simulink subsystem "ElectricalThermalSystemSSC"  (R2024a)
settings: Solver=VariableStepAuto  StartTime=0.0  StopTime=10.0  RelTol=1e-3
undefined symbols (not defined in the file): coolant_pipe_D, coolant_valve_D_ratio_max, coolant_valve_D_ratio_min, coolant_valve_displacement, EnvAirTemp, EnvGrvty, PlantThrEstCmpPwr, PlntThrChArea, PlntThrFanMaxSpd, PlntThrFanMechEff, PlntThrFanVolEff, PlntThrHeaterMaxPwr, PlntThrPipeArea, PlntThrPipeDia, PlntThrPmpMaxSpd, PlntThrRadRamEff, PlntThrRefrigAinit, PlntThrTankArea, PlntThrTankVol, PlntThrValDisp, PlntThrValDratioMax, PlntThrValDratioMin, PlntThrValSplMax, ThrmEM1, ThrmEM2, ThrmEM3, ThrmEM4
libraries: fl_lib x148, nesl_utility x61, SimscapeFluids_lib x25, autolibutils x12
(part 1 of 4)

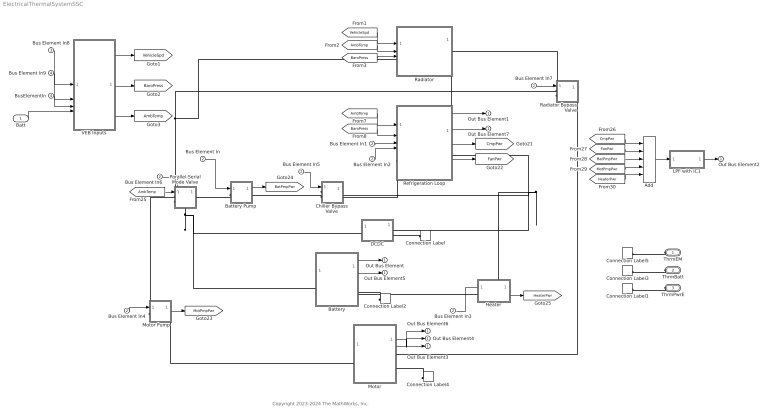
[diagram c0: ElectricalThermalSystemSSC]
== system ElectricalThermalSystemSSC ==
  note: Copyright 2023-2024 The MathWorks, Inc.
  Batt : Inport
  Bus Element In{,1..7} (8 alike) : Inport  Port=2
  Bus Element In8 : Inport  Port=3
  Bus Element In9 : Inport  Port=4
  BusElementIn : Inport  Port=4
  Add : Sum  Inputs=+++++
  Battery : Subsystem  Tag=PublishSubsystem
  Battery Pump : Subsystem  Tag=PublishSubsystem
  Chiller Bypass Valve : Subsystem  Tag=PublishSubsystem
  Connection Label : ConnectionLabel  Label=ThrmPwrE
  Connection Label1 : ConnectionLabel  Label=ThrmPwrE
  Connection Label2 : ConnectionLabel  Label=ThrmBatt
  Connection Label3 : ConnectionLabel  Label=ThrmBatt
  Connection Label4 : ConnectionLabel  Label=ThrmEM
  Connection Label5 : ConnectionLabel  Label=ThrmEM
  DCDC : Subsystem  Tag=PublishSubsystem
  Heater : Subsystem  Tag=PublishSubsystem
  LPF with IC1 : Subsystem  mask{wc=10, InitCond=0, dataType=off}
      mask prompts: wc "Cutoff frequency, wc [rad/s]"; InitCond "Initial condition, InitCond [same as u]"; dataType "Enforce same input data type"
  Motor : Subsystem  Tag=PublishSubsystem
  Motor Pump : Subsystem  Tag=PublishSubsystem
  Parallel-Serial Mode Valve : Subsystem  Tag=PublishSubsystem
  Radiator : Subsystem  Tag=PublishSubsystem
  Radiator Bypass Valve : Subsystem  Tag=PublishSubsystem
  Refrigeration Loop : Subsystem  Tag=detailed cycle  Variant=on  VariantControlMode=label  VariantControl=Choice  LabelModeActiveChoice=System Level
  VEB Inputs : Subsystem
  ThrmEM : PMIOPort  Side=Left
  ThrmBatt : PMIOPort  Port=2  Side=Left
  ThrmPwrE : PMIOPort  Port=3  Side=Left
  Out Bus Element{,1..7} (8 alike) : Outport
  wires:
  Add/1 -> LPF with IC1/1(u)
  Battery/1(01) -> Out Bus Element/1
  [VehicleSpd] -> Radiator/1(1)
  [AmbTemp] -> Radiator/2(2)
  [BaroPress] -> Radiator/3(3)
  [AmbTemp] -> Refrigeration Loop/1(AmbTemp)
  [BaroPress] -> Refrigeration Loop/2(BaroPress)
  Refrigeration Loop/1(CondPress) -> Out Bus Element1/1
  Bus Element In1/1 -> Refrigeration Loop/3(CmpCmd)
  Refrigeration Loop/2(ChlrPress) -> Out Bus Element7/1
  Motor/1(01) -> Out Bus Element4/1, Out Bus Element6/1
  Battery/2(02) -> Out Bus Element5/1
  Bus Element In2/1 -> Refrigeration Loop/4(FanCmd)
  Bus Element In3/1 -> Heater/1(1)
  Bus Element In4/1 -> Motor Pump/1(1)
  Bus Element In/1 -> Battery Pump/1(1)
  Bus Element In5/1 -> Chiller Bypass Valve/1(1)
  Bus Element In6/1 -> Parallel-Serial Mode Valve/2(2)
  Bus Element In7/1 -> Radiator Bypass Valve/1(1)
  [AmbTemp] -> Parallel-Serial Mode Valve/1(1)
  Batt/1 -> VEB Inputs/4(Batt)
  VEB Inputs/1(VehicleSpd) -> [VehicleSpd]
  VEB Inputs/3(AmbTemp) -> [AmbTemp]
  VEB Inputs/2(BaroPress) -> [BaroPress]
  Refrigeration Loop/3(CmpPwr) -> [CmpPwr]
  Refrigeration Loop/4(FanPwr) -> [FanPwr]
  Motor Pump/1(2) -> [MotPmpPwr]
  Battery Pump/1(2) -> [BatPmpPwr]
  [CmpPwr] -> Add/1
  [FanPwr] -> Add/2
  [BatPmpPwr] -> Add/3
  [MotPmpPwr] -> Add/4
  LPF with IC1/1(y) -> Out Bus Element2/1
  Heater/1(2) -> [HeaterPwr]
  [HeaterPwr] -> Add/5
  Motor/2(02) -> Out Bus Element3/1
  Bus Element In8/1 -> VEB Inputs/1(VehBody)
  Bus Element In9/1 -> VEB Inputs/2(Press)
  BusElementIn/1 -> VEB Inputs/3(Temp)
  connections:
  Chiller Bypass Valve/RConn1 -- Heater/RConn1 -- DCDC/RConn1 -- Refrigeration Loop/RConn1
  Parallel-Serial Mode Valve/RConn2 -- Battery/LConn1 -- DCDC/LConn1
  Parallel-Serial Mode Valve/LConn2 -- Radiator/LConn1 -- Radiator Bypass Valve/LConn1
  Connection Label/LConn1 -- DCDC/RConn2
  ThrmPwrE/RConn1 -- Connection Label1/LConn1
  Connection Label2/LConn1 -- Battery/RConn2
  ThrmBatt/RConn1 -- Connection Label3/LConn1
  Connection Label4/LConn1 -- Motor/RConn2
  ThrmEM/RConn1 -- Connection Label5/LConn1
  Battery/RConn1 -- Heater/LConn1
  Motor Pump/RConn1 -- Motor/LConn1
  Radiator Bypass Valve/RConn1 -- Motor/RConn1
  Radiator Bypass Valve/LConn2 -- Radiator/RConn1
  Chiller Bypass Valve/LConn1 -- Battery Pump/RConn1
  Refrigeration Loop/LConn1 -- Chiller Bypass Valve/LConn2
  Battery Pump/LConn1 -- Parallel-Serial Mode Valve/RConn1
  Radiator/RConn2 -- Refrigeration Loop/LConn2
  Motor Pump/LConn1 -- Parallel-Serial Mode Valve/LConn1

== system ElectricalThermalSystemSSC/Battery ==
  Batt Cool1 : fl_lib/Thermal/Thermal Elements/Thermal Mass  mass_type=foundation.enum.constant_variable.constant  mass=1 kg  sp_heat=PlntBattCp J/(K*kg)  mass_min=1e-6 kg  num_ports=foundation.enum.numPorts2.two  m_specify=off  m_priority=High  m=1 kg  m_nominal_specify=off  m_nominal_value=1  m_nominal_unit=kg  T_specify=on  T_priority=High  T=EnvAirTemp K  T_nominal_specify=off  T_nominal_value=1  T_nominal_unit=K  Q_specify=off  Q_priority=None  Q=0 W  Q_nominal_specify=off  Q_nominal_value=1  Q_nominal_unit=W
  Coolant Jacket 1 : SimscapeFluids_lib/Thermal Liquid/Pipes & Fittings/Pipe (TL)  dynamic_compressibility=simscape.enum.onoff.on  inertia=simscape.enum.onoff.off  num_segments=1  pipe_length=PlntThrBattJacLen m  cross_section_geometry=fluids.thermal_liquid.pipes_fittings.enum.CrossSectionGeometry.Custom  pipe_diameter=0.1 m  pipe_inner_diameter=0.05 m  pipe_outer_diameter=0.1 m  pipe_width=0.1 m  pipe_height=0.1 m  pipe_major_axis=0.1 m  pipe_minor_axis=0.05 m  pipe_side=0.1 m  pipe_angle=30 deg  area=4*PlntThrChArea m^2  Dh=PlntThrChDia m  elevation_spec=foundation.enum.constant_variable.constant  elevation_gain=0 m  gravity_spec=foundation.enum.constant_variable.constant  g=EnvGrvty m/s^2  pressure_loss_spec=fluids.thermal_liquid.pipes_fittings.enum.PressureLossSpec.Haaland  local_pressure_loss_spec=fluids.thermal_liquid.pipes_fittings.enum.LocalLossSpec.AggregateLength  length_add=0 m  loss_coefficient=0.1  roughness_spec=fluids.thermal_liquid.pipes_fittings.enum.RoughnessSpec.Custom  roughness=1.5e-5 m  Re_friction_TLU=[ 400 1000 1.5e+3 3e+3 4e+3 6e+3 1e+4 2e+4 4e+4 6e+4 1e+5 1e+8 ]  friction_factor_TLU=[ 0.264 0.112 0.07099999999999999 0.0417 0.0387 0.0268 0.025 0.0232 0.0226 0.022 0.0214 0.0214 ]  Re_lam=100  Re_tur=500  shape_factor=64  mdot_nominal=[ 0.1 1 ] kg/s  p_diff_nominal=[ 0.001 0.01 ] MPa  mdot_threshold=1e-6 kg/s  wall_spec=fluids.thermal_liquid.pipes_fittings.enum.wall_spec.rigid  vol_expansion_spec=fluids.thermal_liquid.pipes_fittings.enum.VolumeExpansionSpec.Diameter  area_pressure_gain=1e-6 m^2/MPa  static_pressure_TLU=[.1, 1] MPa  area_pressure_gain_TLU=[1e-05, 1.1e-05] m^2  material_behavior_spec=fluids.thermal_liquid.pipes_fittings.enum.PipeMaterialBehavior.Linear  diameter_pressure_gain=1.2e-6 m/MPa  wall_thickness=0.05 m  elastic_modulus=69 GPa  stress_TLU=[276, 310] MPa  strain_TLU=[.004, .02]  stress_assert_action=simscape.enum.assert.action.none  stress_max=400 MPa  poisson_ratio=0.33  wall_time_constant=0.01 s  thermal_expansion=false  alpha_L_wall=24 um/(deltaK*m)  thermal_expansion_Tref=293.15 K  heat_transfer_spec=fluids.thermal_liquid.pipes_fittings.enum.HeatTransferSpec.DittusBoelter  mdot_nominal_heat=[ 0.1 1 ] kg/s  T_in_nominal=[ 293.15 293.15 ] K  T_out_nominal=[ 300 300 ] K  p_in_nominal_heat=[ 0.101325 0.101325 ] MPa  T_wall_nominal=[ 303.15 303.15 ] K  a_coeff=0.3  b_Re_power=0.8  c_Pr_power=0.33  Nu_lam=3.66  Re_Colburn_TLU=[ 100 150 1000 ]  Colburn_factor_TLU=[ 0.019 0.013 0.002 ]  Re_Nu_TLU=[ 100 150 1000 ]  Pr_Nu_TLU=[ 1 10 ]  Nu_TLU=[ 3.72 4.21; 3.75 4.44; 4.21 7.15 ]  p0_vec=EnvAbsPrs Pa  T0_vec=EnvAirTemp K  mdot0=0.1 kg/s
  Flow Resistance (TL) : fl_lib/Thermal Liquid/Elements/Flow Resistance (TL)  delta_p_nominal=200 Pa  mdot_nominal=0.02 kg/s  area=PlntThrPipeArea m^2  laminar_fraction=1e-3
  S1 : Subsystem
  SC1 : Subsystem
  SC2 : Subsystem
  Simscape Bus2 : SimscapeBus  HierarchyStrings=ThrmBatt1
  B : PMIOPort  Side=Left
  A : PMIOPort  Port=2  Side=Right
  T : PMIOPort  Port=3  Side=Right
  01 : Outport
  02 : Outport  Port=2
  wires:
  S1/1(BattTemp) -> 02/1
  SC1/1(BattCoolTemp) -> 01/1
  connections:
  Batt Cool1/LConn1 -- S1/RConn1
  Batt Cool1/RConn1 -- Simscape Bus2/LConn1
  S1/LConn1 -- Coolant Jacket 1/LConn2
  SC1/LConn1 -- Coolant Jacket 1/LConn1
  A/RConn1 -- SC1/RConn1
  SC2/RConn1 -- Coolant Jacket 1/RConn1
  SC2/LConn1 -- Flow Resistance (TL)/LConn1
  Flow Resistance (TL)/RConn1 -- B/RConn1
  T/RConn1 -- Simscape Bus2/RConn1

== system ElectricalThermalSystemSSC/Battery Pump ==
  1 : Inport
  Battery Pump : SimscapeFluids_lib/Thermal Liquid/Pumps & Motors/Fixed-Displacement Pump (TL)  loss_spec=fluids.thermal_liquid.pumps_motors.enum.LossSpec.TabulatedEfficiency  displacement=PlntThrPmpDisp l/rev  omega_nominal=0.5 * PlntThrPmpMaxSpd rpm  p_nominal=0.1 MPa  mu_nominal=0.9 cP  vol_eff_nominal=PlntThrPmpVolEff  mech_eff_nominal=PlntThrPmpMechEff  no_load_torque=0.03 N*m  p_diff_eff_TLU=[.1, 1, 2] MPa  omega_eff_TLU=[25, 50, 100, 200, 300, 400] rad/s  vol_eff_TLU=[.816, .908, .954, .977, .981, .984; .325, .663, .831, .916, .925, .946; .137, .568, .78, .892, .893, .91]  mech_eff_TLU=[.996, .996, .996, .996, .996, .996; .988, .989, .989, .989, .989, .99; .981, .981, .982, .982, .983, .984]  p_diff_loss_TLU=[.1, 1, 2] MPa  omega_loss_TLU=[25, 50, 100, 200, 300, 400] rad/s  vol_loss_TLU=[.023, .023, .023, .023, .0285, .032; .0844, .0842, .0845, .084, .1125, .108; .1079, .108, .11, .108, .1605, .18] * 1e-3 m^3/s  mech_loss_TLU=[.002, .002, .002, .002, .002, .002; .0607, .0556, .0556, .0556, .0556, .0505; .1937, .1937, .1833, .1833, .1729, .1626] N*m  vol_eff_min=1e-3  vol_eff_max=1  mech_eff_min=1e-3  mech_eff_max=1  pressure_threshold=1e-3 MPa  omega_threshold=10 rad/s  area=PlntThrPipeArea m^2  supplied_range_check=0  pump_mode_check=simscape.enum.assert.action.none
  Ideal Angular Velocity Source : fl_lib/Mechanical/Mechanical Sources/Ideal Angular Velocity Source
  Ideal Rotational Motion Sensor : fl_lib/Mechanical/Mechanical Sensors/Ideal Rotational Motion Sensor  reference=foundation.enum.MeasurementReference.difference  acceleration_port=false  velocity_port=true  position_port=true  wrap_angle=false  offset=0 rad
  Ideal Torque Sensor : fl_lib/Mechanical/Mechanical Sensors/Ideal Torque Sensor
  LPF with IC1 : Subsystem  mask{wc=0.2, InitCond=0, dataType=off}
      mask prompts: wc "Cutoff frequency, wc [rad/s]"; InitCond "Initial condition, InitCond [same as u]"; dataType "Enforce same input data type"
  Max Speed [rpm] : Gain  Gain=PlntThrPmpMaxSpd
  Mechanical Rotational Reference : fl_lib/Mechanical/Rotational Elements/Mechanical Rotational Reference
  Mechanical Rotational Reference1 : fl_lib/Mechanical/Rotational Elements/Mechanical Rotational Reference
  PS Product : fl_lib/Physical Signals/Functions/PS Product
  PS-Simulink Converter : nesl_utility/PS-Simulink Converter  PhysicalDomain=network_engine_domain  SubClassName=ps_output  LeftPortType=input  RightPortType=output  PseudoPeriodic=off  Frequencies=[]  VectorFormat=inherit  Unit=W  AffineConversion=off
  Simulink-PS Converter : nesl_utility/Simulink-PS Converter  PhysicalDomain=network_engine_domain  SubClassName=ps_input  LeftPortType=input  RightPortType=output  PseudoPeriodic=off  Frequencies=[]  NoiseDistribution=none  NoiseParameters=[]  Unit=rpm  AffineConversion=off  FilteringAndDerivatives=provide  SimscapeFilterOrder=1  InputFilterTimeConstant=0.001  UdotUserProvided=0
  A : PMIOPort  Side=Left
  B : PMIOPort  Port=2  Side=Right
  2 : Outport
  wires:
  PS-Simulink Converter/1 -> 2/1
  Max Speed [rpm]/1 -> Simulink-PS Converter/1
  1/1 -> LPF with IC1/1(u)
  LPF with IC1/1(y) -> Max Speed [rpm]/1
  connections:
  Ideal Rotational Motion Sensor/LConn1 -- Ideal Angular Velocity Source/LConn1 -- Ideal Torque Sensor/LConn1
  Ideal Torque Sensor/RConn1 -- Battery Pump/RConn1
  PS Product/LConn1 -- Ideal Rotational Motion Sensor/RConn2
  PS-Simulink Converter/LConn1 -- PS Product/RConn1
  PS Product/LConn2 -- Ideal Torque Sensor/RConn2
  Mechanical Rotational Reference1/LConn1 -- Ideal Rotational Motion Sensor/RConn1
  Battery Pump/LConn2 -- B/RConn1
  Battery Pump/LConn1 -- A/RConn1
  Battery Pump/RConn2 -- Mechanical Rotational Reference/LConn1 -- Ideal Angular Velocity Source/RConn2
  Simulink-PS Converter/RConn1 -- Ideal Angular Velocity Source/RConn1

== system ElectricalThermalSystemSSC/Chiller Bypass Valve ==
  1 : Inport
  Bias : Bias  Bias=-1
  Chiller Bypass Valve : SimscapeFluids_lib/Thermal Liquid/Valves & Orifices/Directional Control Valves/3-Way Directional Valve (TL)  open_orifices_pos=fluids.thermal_liquid.valves.directional_control_valves.enum.OpenOrifices3Way.PA  open_orifices_neg=fluids.thermal_liquid.valves.directional_control_valves.enum.OpenOrifices3Way.AT  area_spec=fluids.thermal_liquid.valves.directional_control_valves.enum.area_spec.identical  valve_spec=fluids.thermal_liquid.valves.enum.orifice_spec.linear  del_S_max=PlntThrValDisp m  area_max=pi * (PlntThrValDratioMax*PlntThrPipeDia)^2 / 4 m^2  del_S_TLU=[0 0.002 0.004 0.007 0.017] m  valve_area_TLU=[1e-09, 2.0352e-07, 4.0736e-05, .00011438, .00034356] m^2  del_S_flow_TLU=[0 0.002 0.004 0.007 0.017] m  p_diff_TLU=[-.1, .3, .5, .7] MPa  vol_flow_TLU=1e-3 * [1.7e-05, 2e-05, 2.6e-05; .0035, .0045, .0053; .7, .9, 1.06; 1.96, 2.5, 3; 6, 7.7, 9.13] m^3/s  mdot_TLU=[-1e-05, 1.7e-05, 2e-05, 2.6e-05; -.002, .0035, .0045, .0053; -.4, .7, .9, 1.06; -1.13, 1.96, 2.5, 3; -3.45, 6, 7.7, 9.13] kg/s  T_ref_in=293.15 K  p_ref_in=0.101325 MPa  area_leak=pi * (PlntThrValDratioMin*PlntThrPipeDia)^2 / 4 m^2  Cd=0.7  Re_c=12  smoothing_factor=0.01  pressure_recovery=simscape.enum.onoff.on  area=pi *PlntThrPipeDia^2 / 4 m^2  S_max_PA=PlntThrValSplMax m  del_S_max_PA=coolant_valve_displacement-(coolant_valve_displacement)*(pi * (coolant_valve_D_ratio_min*coolant_pipe_D)^2 / 4)/(pi * (coolant_valve_D_ratio_max*coolant_pipe_D)^2 / 4) m  area_max_PA=pi * (coolant_valve_D_ratio_max*coolant_pipe_D)^2 / 4 m^2  del_S_TLU_PA=[0 0.002 0.004 0.007 0.017] m  valve_area_TLU_PA=[1e-09, 2.0352e-07, 4.0736e-05, .00011438, .00034356] m^2  del_S_flow_TLU_PA=[0 0.002 0.004 0.007 0.017] m  p_diff_TLU_PA=[-.1, .3, .5, .7] MPa  vol_flow_TLU_PA=1e-3 * [1.7e-05, 2e-05, 2.6e-05; .0035, .0045, .0053; .7, .9, 1.06; 1.96, 2.5, 3; 6, 7.7, 9.13] m^3/s  mdot_TLU_PA=[-1e-05, 1.7e-05, 2e-05, 2.6e-05; -.002, .0035, .0045, .0053; -.4, .7, .9, 1.06; -1.13, 1.96, 2.5, 3; -3.45, 6, 7.7, 9.13] kg/s  S_max_AT=-PlntThrValSplMax m  del_S_max_AT=coolant_valve_displacement-(coolant_valve_displacement)*(pi * (coolant_valve_D_ratio_min*coolant_pipe_D)^2 / 4)/(pi * (coolant_valve_D_ratio_max*coolant_pipe_D)^2 / 4) m  area_max_AT=pi * (coolant_valve_D_ratio_max*coolant_pipe_D)^2 / 4 m^2  del_S_TLU_AT=[0 0.002 0.004 0.007 0.017] m  valve_area_TLU_AT=[1e-09, 2.0352e-07, 4.0736e-05, .00011438, .00034356] m^2  del_S_flow_TLU_AT=[0 0.002 0.004 0.007 0.017] m  p_diff_TLU_AT=[-.1, .3, .5, .7] MPa  vol_flow_TLU_AT=1e-3 * [1.7e-05, 2e-05, 2.6e-05; .0035, .0045, .0053; .7, .9, 1.06; 1.96, 2.5, 3; 6, 7.7, 9.13] m^3/s  mdot_TLU_AT=[-1e-05, 1.7e-05, 2e-05, 2.6e-05; -.002, .0035, .0045, .0053; -.4, .7, .9, 1.06; -1.13, 1.96, 2.5, 3; -3.45, 6, 7.7, 9.13] kg/s  S_max_PT=2.5e-3 m  del_S_max_PT=0.005 m  area_max_PT=1e-4 m^2  del_S_TLU_PT=[0, .002, .004, .007, .017] m  valve_area_TLU_PT=[1e-09, 2.0352e-07, 4.0736e-05, .00011438, .00034356] m^2  del_S_flow_TLU_PT=[0, .002, .004, .007, .017] m  p_diff_TLU_PT=[.3, .5, .7] MPa  vol_flow_TLU_PT=1e-3 * [1.7e-05, 2e-05, 2.6e-05; .0035, .0045, .0053; .7, .9, 1.06; 1.96, 2.5, 3; 6, 7.7, 9.13] m^3/s  mdot_TLU_PT=[1.7e-05, 2e-05, 2.6e-05; .0035, .0045, .0053; .7, .9, 1.06; 1.96, 2.5, 3; 6, 7.7, 9.13] kg/s
  Flow Resistance (TL) : fl_lib/Thermal Liquid/Elements/Flow Resistance (TL)  delta_p_nominal=0.001 MPa  mdot_nominal=0.3 kg/s  area=pi * PlntThrPipeDia^2 / 4 m^2  laminar_fraction=1e-3
  Gain : Gain  Gain=2
  LPF with IC1 : Subsystem  mask{wc=1, InitCond=0, dataType=off}
      mask prompts: wc "Cutoff frequency, wc [rad/s]"; InitCond "Initial condition, InitCond [same as u]"; dataType "Enforce same input data type"
  Max Valve Displacement [m] : Gain  Gain=PlntThrValDisp
  Simulink-PS Converter : nesl_utility/Simulink-PS Converter  PhysicalDomain=network_engine_domain  SubClassName=ps_input  LeftPortType=input  RightPortType=output  PseudoPeriodic=off  Frequencies=[]  NoiseDistribution=none  NoiseParameters=[]  Unit=m  AffineConversion=off  FilteringAndDerivatives=provide  SimscapeFilterOrder=1  InputFilterTimeConstant=0.001  UdotUserProvided=0
  A : PMIOPort  Side=Left
  C : PMIOPort  Port=2  Side=Left
  B : PMIOPort  Port=3  Side=Right
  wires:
  1/1 -> LPF with IC1/1(u)
  Gain/1 -> Bias/1
  Bias/1 -> Max Valve Displacement [m]/1
  Max Valve Displacement [m]/1 -> Simulink-PS Converter/1
  LPF with IC1/1(y) -> Gain/1
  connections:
  Flow Resistance (TL)/RConn1 -- B/RConn1
  Chiller Bypass Valve/RConn2 -- Flow Resistance (TL)/LConn1
  Chiller Bypass Valve/RConn1 -- Simulink-PS Converter/RConn1
  Chiller Bypass Valve/RConn3 -- C/RConn1
  Chiller Bypass Valve/LConn1 -- A/RConn1

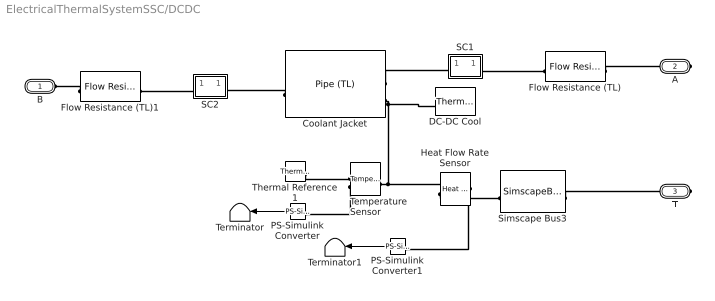
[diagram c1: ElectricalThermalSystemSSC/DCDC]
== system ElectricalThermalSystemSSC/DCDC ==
  Coolant Jacket : SimscapeFluids_lib/Thermal Liquid/Pipes & Fittings/Pipe (TL)  dynamic_compressibility=simscape.enum.onoff.on  inertia=simscape.enum.onoff.off  num_segments=1  pipe_length=PlntThrDCJacLen m  cross_section_geometry=fluids.thermal_liquid.pipes_fittings.enum.CrossSectionGeometry.Custom  pipe_diameter=0.1 m  pipe_inner_diameter=0.05 m  pipe_outer_diameter=0.1 m  pipe_width=0.1 m  pipe_height=0.1 m  pipe_major_axis=0.1 m  pipe_minor_axis=0.05 m  pipe_side=0.1 m  pipe_angle=30 deg  area=PlntThrChArea m^2  Dh=PlntThrChDia m  elevation_spec=foundation.enum.constant_variable.constant  elevation_gain=0 m  gravity_spec=foundation.enum.constant_variable.constant  g=EnvGrvty m/s^2  pressure_loss_spec=fluids.thermal_liquid.pipes_fittings.enum.PressureLossSpec.Haaland  local_pressure_loss_spec=fluids.thermal_liquid.pipes_fittings.enum.LocalLossSpec.AggregateLength  length_add=0 m  loss_coefficient=0.1  roughness_spec=fluids.thermal_liquid.pipes_fittings.enum.RoughnessSpec.Custom  roughness=1.5e-5 m  Re_friction_TLU=[ 400 1000 1.5e+3 3e+3 4e+3 6e+3 1e+4 2e+4 4e+4 6e+4 1e+5 1e+8 ]  friction_factor_TLU=[ 0.264 0.112 0.07099999999999999 0.0417 0.0387 0.0268 0.025 0.0232 0.0226 0.022 0.0214 0.0214 ]  Re_lam=100  Re_tur=500  shape_factor=64  mdot_nominal=[ 0.1 1 ] kg/s  p_diff_nominal=[ 0.001 0.01 ] MPa  mdot_threshold=1e-6 kg/s  wall_spec=fluids.thermal_liquid.pipes_fittings.enum.wall_spec.rigid  vol_expansion_spec=fluids.thermal_liquid.pipes_fittings.enum.VolumeExpansionSpec.Diameter  area_pressure_gain=1e-6 m^2/MPa  static_pressure_TLU=[.1, 1] MPa  area_pressure_gain_TLU=[1e-05, 1.1e-05] m^2  material_behavior_spec=fluids.thermal_liquid.pipes_fittings.enum.PipeMaterialBehavior.Linear  diameter_pressure_gain=1.2e-6 m/MPa  wall_thickness=0.05 m  elastic_modulus=69 GPa  stress_TLU=[276, 310] MPa  strain_TLU=[.004, .02]  stress_assert_action=simscape.enum.assert.action.none  stress_max=400 MPa  poisson_ratio=0.33  wall_time_constant=0.01 s  thermal_expansion=false  alpha_L_wall=24 um/(deltaK*m)  thermal_expansion_Tref=293.15 K  heat_transfer_spec=fluids.thermal_liquid.pipes_fittings.enum.HeatTransferSpec.DittusBoelter  mdot_nominal_heat=[ 0.1 1 ] kg/s  T_in_nominal=[ 293.15 293.15 ] K  T_out_nominal=[ 300 300 ] K  p_in_nominal_heat=[ 0.101325 0.101325 ] MPa  T_wall_nominal=[ 303.15 303.15 ] K  a_coeff=0.3  b_Re_power=0.8  c_Pr_power=0.33  Nu_lam=3.66  Re_Colburn_TLU=[ 100 150 1000 ]  Colburn_factor_TLU=[ 0.019 0.013 0.002 ]  Re_Nu_TLU=[ 100 150 1000 ]  Pr_Nu_TLU=[ 1 10 ]  Nu_TLU=[ 3.72 4.21; 3.75 4.44; 4.21 7.15 ]  p0_vec=EnvAbsPrs Pa  T0_vec=EnvAirTemp K  mdot0=0.1 kg/s
  DC-DC Cool : fl_lib/Thermal/Thermal Elements/Thermal Mass  mass_type=foundation.enum.constant_variable.constant  mass=1 kg  sp_heat=PlntEMCp J/(K*kg)  mass_min=1e-6 kg  num_ports=foundation.enum.numPorts2.one  m_specify=off  m_priority=High  m=1 kg  m_nominal_specify=off  m_nominal_value=1  m_nominal_unit=kg  T_specify=on  T_priority=High  T=EnvAirTemp K  T_nominal_specify=off  T_nominal_value=1  T_nominal_unit=K  Q_specify=off  Q_priority=None  Q=0 W  Q_nominal_specify=off  Q_nominal_value=1  Q_nominal_unit=W
  Flow Resistance (TL) : fl_lib/Thermal Liquid/Elements/Flow Resistance (TL)  delta_p_nominal=2e-3 MPa  mdot_nominal=0.02 kg/s  area=PlntThrPipeArea m^2  laminar_fraction=1e-3
  Flow Resistance (TL)1 : fl_lib/Thermal Liquid/Elements/Flow Resistance (TL)  delta_p_nominal=1e-5 MPa  mdot_nominal=0.02 kg/s  area=PlntThrPipeArea m^2  laminar_fraction=1e-3
  Heat Flow Rate Sensor : fl_lib/Thermal/Thermal Sensors/Heat Flow Rate Sensor
  PS-Simulink Converter : nesl_utility/PS-Simulink Converter  PhysicalDomain=network_engine_domain  SubClassName=ps_output  LeftPortType=input  RightPortType=output  PseudoPeriodic=off  Frequencies=[]  VectorFormat=1-D array  Unit=K  AffineConversion=on
  PS-Simulink Converter1 : nesl_utility/PS-Simulink Converter  PhysicalDomain=network_engine_domain  SubClassName=ps_output  LeftPortType=input  RightPortType=output  PseudoPeriodic=off  Frequencies=[]  VectorFormat=1-D array  Unit=J/s  AffineConversion=off
  SC1 : Subsystem
  SC2 : Subsystem
  Simscape Bus3 : SimscapeBus  HierarchyStrings=ThrmPwrE1
  Temperature Sensor : fl_lib/Thermal/Thermal Sensors/Temperature Sensor  temperature_measure=foundation.enum.MeasurementReference.difference
  Terminator : Terminator
  Terminator1 : Terminator
  Thermal Reference1 : fl_lib/Thermal/Thermal Elements/Thermal Reference
  B : PMIOPort  Side=Left
  A : PMIOPort  Port=2  Side=Right
  T : PMIOPort  Port=3  Side=Right
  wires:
  PS-Simulink Converter1/1 -> Terminator1/1
  PS-Simulink Converter/1 -> Terminator/1
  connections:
  Heat Flow Rate Sensor/RConn1 -- PS-Simulink Converter1/LConn1
  Heat Flow Rate Sensor/LConn1 -- Simscape Bus3/LConn1
  Temperature Sensor/LConn1 -- Heat Flow Rate Sensor/RConn2 -- DC-DC Cool/LConn1 -- Coolant Jacket/LConn2
  Thermal Reference1/LConn1 -- Temperature Sensor/RConn1
  Temperature Sensor/RConn2 -- PS-Simulink Converter/LConn1
  SC1/RConn1 -- Flow Resistance (TL)/RConn1
  SC2/LConn1 -- Flow Resistance (TL)1/LConn1
  Flow Resistance (TL)/LConn1 -- A/RConn1
  Flow Resistance (TL)1/RConn1 -- B/RConn1
  Coolant Jacket/LConn1 -- SC1/LConn1
  Coolant Jacket/RConn1 -- SC2/RConn1
  Simscape Bus3/RConn1 -- T/RConn1

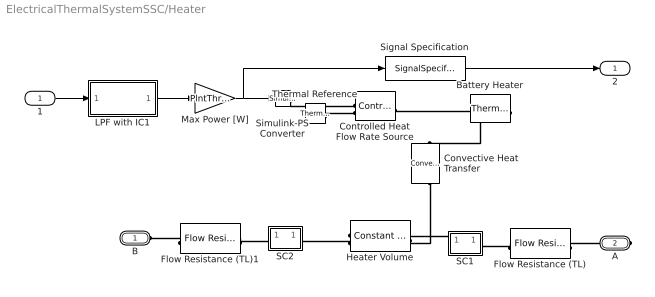
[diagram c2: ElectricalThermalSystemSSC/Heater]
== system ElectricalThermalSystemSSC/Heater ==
  1 : Inport
  Battery Heater : fl_lib/Thermal/Thermal Elements/Thermal Mass  mass_type=foundation.enum.constant_variable.constant  mass=2 kg  sp_heat=447 J/kg/K  mass_min=1e-6 kg  num_ports=foundation.enum.numPorts2.one  m_specify=off  m_priority=High  m=1 kg  m_nominal_specify=off  m_nominal_value=1  m_nominal_unit=kg  T_specify=on  T_priority=High  T=EnvAirTemp K  T_nominal_specify=off  T_nominal_value=1  T_nominal_unit=K  Q_specify=off  Q_priority=None  Q=0 W  Q_nominal_specify=off  Q_nominal_value=1  Q_nominal_unit=W
  Controlled Heat Flow Rate Source : fl_lib/Thermal/Thermal Sources/Controlled Heat Flow Rate Source
  Convective Heat Transfer : fl_lib/Thermal/Thermal Elements/Convective Heat Transfer  thermal_type=foundation.enum.constant_variable.constant  area=PlntThrHeaterJacArea m^2  heat_tr_coeff=PlntThrHeaterCoeff W/(m^2 * K)  min_heat_tr_coeff=1e-3 W/(K*m^2)  T_specify=off  T_priority=None  T=0 K  T_nominal_specify=off  T_nominal_value=1  T_nominal_unit=K  Q_specify=off  Q_priority=None  Q=0 W  Q_nominal_specify=off  Q_nominal_value=1  Q_nominal_unit=W
  Flow Resistance (TL) : fl_lib/Thermal Liquid/Elements/Flow Resistance (TL)  delta_p_nominal=2e-4 MPa  mdot_nominal=0.15 kg/s  area=PlntThrPipeArea m^2  laminar_fraction=1e-3
  Flow Resistance (TL)1 : fl_lib/Thermal Liquid/Elements/Flow Resistance (TL)  delta_p_nominal=2e-4 MPa  mdot_nominal=0.15 kg/s  area=PlntThrPipeArea m^2  laminar_fraction=1e-3
  Heater Volume : fl_lib/Thermal Liquid/Elements/Constant Volume Chamber (TL)  volume=PlntThrHeaterJacVol m^3  num_ports=foundation.enum.num_ports.two  area_A=PlntThrPipeArea m^2  area_B=PlntThrPipeArea m^2  area_C=0.01 m^2  area_D=0.01 m^2  p_I_specify=on  p_I_priority=High  p_I=EnvAbsPrs Pa  p_I_nominal_specify=off  p_I_nominal_value=1  p_I_nominal_unit=MPa  T_I_specify=on  T_I_priority=High  T_I=EnvAirTemp K  T_I_nominal_specify=off  T_I_nominal_value=1  T_I_nominal_unit=K  u_I_specify=off  u_I_priority=None  u_I=83.90600000000001 kJ/kg  u_I_nominal_specify=off  u_I_nominal_value=1  u_I_nominal_unit=kJ/kg  rho_I_specify=off  rho_I_priority=None  rho_I=998.21 kg/m^3  rho_I_nominal_specify=off  rho_I_nominal_value=1  rho_I_nominal_unit=kg/m^3
  LPF with IC1 : Subsystem  mask{wc=1, InitCond=0, dataType=off}
      mask prompts: wc "Cutoff frequency, wc [rad/s]"; InitCond "Initial condition, InitCond [same as u]"; dataType "Enforce same input data type"
  Max Power [W] : Gain  Gain=PlntThrHeaterMaxPwr
  SC1 : Subsystem
  SC2 : Subsystem
  Signal Specification : SignalSpecification  Unit=W
  Simulink-PS Converter : nesl_utility/Simulink-PS Converter  PhysicalDomain=network_engine_domain  SubClassName=ps_input  LeftPortType=input  RightPortType=output  PseudoPeriodic=off  Frequencies=[]  NoiseDistribution=none  NoiseParameters=[]  Unit=W  AffineConversion=off  FilteringAndDerivatives=provide  SimscapeFilterOrder=1  InputFilterTimeConstant=0.001  UdotUserProvided=0
  Thermal Reference : fl_lib/Thermal/Thermal Elements/Thermal Reference
  B : PMIOPort  Side=Left
  A : PMIOPort  Port=2  Side=Right
  2 : Outport
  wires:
  Max Power [W]/1 -> Signal Specification/1, Simulink-PS Converter/1
  LPF with IC1/1(y) -> Max Power [W]/1
  1/1 -> LPF with IC1/1(u)
  Signal Specification/1 -> 2/1
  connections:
  Flow Resistance (TL)1/RConn1 -- B/RConn1
  Battery Heater/LConn1 -- Convective Heat Transfer/LConn1 -- Controlled Heat Flow Rate Source/LConn1
  Simulink-PS Converter/RConn1 -- Controlled Heat Flow Rate Source/RConn1
  Thermal Reference/LConn1 -- Controlled Heat Flow Rate Source/RConn2
  SC1/LConn1 -- Heater Volume/LConn1
  Flow Resistance (TL)/LConn1 -- A/RConn1
  SC2/RConn1 -- Heater Volume/RConn1
  Convective Heat Transfer/RConn1 -- Heater Volume/LConn2
  Flow Resistance (TL)/RConn1 -- SC1/RConn1
  Flow Resistance (TL)1/LConn1 -- SC2/LConn1

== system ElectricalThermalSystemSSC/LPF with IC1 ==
  u : Inport
  Cont LPF IC : autolibutils/Cont LPF IC  wc=wc  aMode=1  dataType=off
  Initial Condition : Constant  Value=InitCond  SampleTime=-1
  y : Outport
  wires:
  Initial Condition/1 -> Cont LPF IC/2
  u/1 -> Cont LPF IC/1
  Cont LPF IC/1 -> y/1

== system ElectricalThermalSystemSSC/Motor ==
  Cooling Assembly : Subsystem  Variant=on  VariantControl=Cooling Assembly
  PS-Simulink Converter : nesl_utility/PS-Simulink Converter  PhysicalDomain=network_engine_domain  SubClassName=ps_output  LeftPortType=input  RightPortType=output  PseudoPeriodic=off  Frequencies=[]  VectorFormat=inherit  Unit=K  AffineConversion=on
  Pressure & Temperature Sensor (TL) : fl_lib/Thermal Liquid/Sensors/Pressure & Temperature Sensor (TL)  reference=foundation.enum.MeasurementReference.absolute  pressure=false  pressure_spec=foundation.enum.PressureMeasementSpec.Absolute  temperature=true
  Simscape Bus1 : SimscapeBus  HierarchyStrings=ThrmEM4;ThrmEM3;ThrmEM2;ThrmEM1
  A : PMIOPort  Side=Left
  B : PMIOPort  Port=2  Side=Right
  T : PMIOPort  Port=3  Side=Right
  01 : Outport
  02 : Outport  Port=2
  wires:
  PS-Simulink Converter/1 -> 02/1
  Cooling Assembly/1(EMTemp) -> 01/1
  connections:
  PS-Simulink Converter/LConn1 -- Pressure & Temperature Sensor (TL)/RConn1
  Simscape Bus1/LConn1 -- Cooling Assembly/RConn2
  Simscape Bus1/LConn2 -- Cooling Assembly/RConn3
  Simscape Bus1/LConn3 -- Cooling Assembly/RConn4
  Simscape Bus1/LConn4 -- Cooling Assembly/RConn5
  Cooling Assembly/RConn1 -- Pressure & Temperature Sensor (TL)/LConn1 -- B/RConn1
  A/RConn1 -- Cooling Assembly/LConn1
  T/RConn1 -- Simscape Bus1/RConn1

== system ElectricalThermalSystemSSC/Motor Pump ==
  1 : Inport
  Ideal Angular Velocity Source : fl_lib/Mechanical/Mechanical Sources/Ideal Angular Velocity Source
  Ideal Rotational Motion Sensor : fl_lib/Mechanical/Mechanical Sensors/Ideal Rotational Motion Sensor  reference=foundation.enum.MeasurementReference.difference  acceleration_port=false  velocity_port=true  position_port=true  wrap_angle=false  offset=0 rad
  Ideal Torque Sensor : fl_lib/Mechanical/Mechanical Sensors/Ideal Torque Sensor
  LPF with IC1 : Subsystem  mask{wc=0.2, InitCond=0, dataType=off}
      mask prompts: wc "Cutoff frequency, wc [rad/s]"; InitCond "Initial condition, InitCond [same as u]"; dataType "Enforce same input data type"
  Max Speed [rpm] : Gain  Gain=PlntThrPmpMaxSpd
  Mechanical Rotational Reference : fl_lib/Mechanical/Rotational Elements/Mechanical Rotational Reference
  Mechanical Rotational Reference1 : fl_lib/Mechanical/Rotational Elements/Mechanical Rotational Reference
  Motor Pump : SimscapeFluids_lib/Thermal Liquid/Pumps & Motors/Fixed-Displacement Pump (TL)  loss_spec=fluids.thermal_liquid.pumps_motors.enum.LossSpec.TabulatedEfficiency  displacement=PlntThrPmpDisp l/rev  omega_nominal=0.5 * PlntThrPmpMaxSpd rpm  p_nominal=0.1 MPa  mu_nominal=0.9 cP  vol_eff_nominal=PlntThrPmpVolEff  mech_eff_nominal=PlntThrPmpMechEff  no_load_torque=0.03 N*m  p_diff_eff_TLU=[.1, 1, 2] MPa  omega_eff_TLU=[25, 50, 100, 200, 300, 400] rad/s  vol_eff_TLU=[.816, .908, .954, .977, .981, .984; .325, .663, .831, .916, .925, .946; .137, .568, .78, .892, .893, .91]  mech_eff_TLU=[.996, .996, .996, .996, .996, .996; .988, .989, .989, .989, .989, .99; .981, .981, .982, .982, .983, .984]  p_diff_loss_TLU=[.1, 1, 2] MPa  omega_loss_TLU=[25, 50, 100, 200, 300, 400] rad/s  vol_loss_TLU=[.023, .023, .023, .023, .0285, .032; .0844, .0842, .0845, .084, .1125, .108; .1079, .108, .11, .108, .1605, .18] * 1e-3 m^3/s  mech_loss_TLU=[.002, .002, .002, .002, .002, .002; .0607, .0556, .0556, .0556, .0556, .0505; .1937, .1937, .1833, .1833, .1729, .1626] N*m  vol_eff_min=1e-3  vol_eff_max=1  mech_eff_min=1e-3  mech_eff_max=1  pressure_threshold=1e-3 MPa  omega_threshold=10 rad/s  area=PlntThrPipeArea m^2  supplied_range_check=0  pump_mode_check=simscape.enum.assert.action.none
  PS Product : fl_lib/Physical Signals/Functions/PS Product
  PS-Simulink Converter : nesl_utility/PS-Simulink Converter  PhysicalDomain=network_engine_domain  SubClassName=ps_output  LeftPortType=input  RightPortType=output  PseudoPeriodic=off  Frequencies=[]  VectorFormat=inherit  Unit=W  AffineConversion=off
  Simulink-PS Converter : nesl_utility/Simulink-PS Converter  PhysicalDomain=network_engine_domain  SubClassName=ps_input  LeftPortType=input  RightPortType=output  PseudoPeriodic=off  Frequencies=[]  NoiseDistribution=none  NoiseParameters=[]  Unit=rpm  AffineConversion=off  FilteringAndDerivatives=provide  SimscapeFilterOrder=1  InputFilterTimeConstant=0.001  UdotUserProvided=0
  A : PMIOPort  Side=Left
  B : PMIOPort  Port=2  Side=Right
  2 : Outport
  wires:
  PS-Simulink Converter/1 -> 2/1
  Max Speed [rpm]/1 -> Simulink-PS Converter/1
  LPF with IC1/1(y) -> Max Speed [rpm]/1
  1/1 -> LPF with IC1/1(u)
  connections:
  Ideal Rotational Motion Sensor/LConn1 -- Ideal Angular Velocity Source/LConn1 -- Ideal Torque Sensor/LConn1
  Motor Pump/RConn1 -- Ideal Torque Sensor/RConn1
  PS Product/RConn1 -- PS-Simulink Converter/LConn1
  Mechanical Rotational Reference1/LConn1 -- Ideal Rotational Motion Sensor/RConn1
  PS Product/LConn1 -- Ideal Rotational Motion Sensor/RConn2
  PS Product/LConn2 -- Ideal Torque Sensor/RConn2
  Motor Pump/LConn2 -- B/RConn1
  Motor Pump/LConn1 -- A/RConn1
  Ideal Angular Velocity Source/RConn2 -- Motor Pump/RConn2 -- Mechanical Rotational Reference/LConn1
  Simulink-PS Converter/RConn1 -- Ideal Angular Velocity Source/RConn1

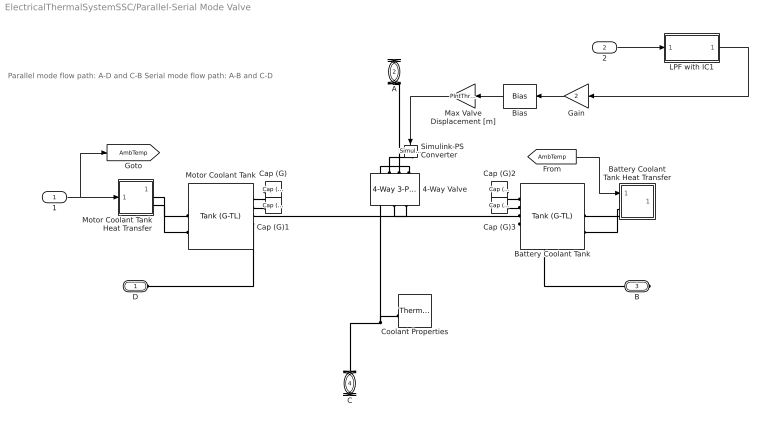
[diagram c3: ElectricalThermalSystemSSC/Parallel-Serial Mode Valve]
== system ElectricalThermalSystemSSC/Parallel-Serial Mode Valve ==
  note: Parallel mode flow path: A-D and C-B Serial mode flow path: A-B and C-D
  1 : Inport
  2 : Inport  Port=2
  4-Way Valve : SimscapeFluids_lib/Thermal Liquid/Valves & Orifices/Directional Control Valves/4-Way 3-Position Directional Valve (TL)  open_orifices_pos=fluids.thermal_liquid.valves.directional_control_valves.enum.OpenOrifices4WayPosNeg.PA_BT  open_orifices_neu=fluids.thermal_liquid.valves.directional_control_valves.enum.OpenOrifices4WayNeu.all_closed  open_orifices_neg=fluids.thermal_liquid.valves.directional_control_valves.enum.OpenOrifices4WayPosNeg.PB_AT  neutral_assert_action=simscape.enum.assert.action.none  area_spec=fluids.thermal_liquid.valves.directional_control_valves.enum.area_spec.identical  valve_spec=fluids.thermal_liquid.valves.enum.orifice_spec.linear  del_S_max=PlntThrValDisp m  area_max=pi * (PlntThrValDratioMax*PlntThrPipeDia)^2 / 4 m^2  del_S_TLU=[0 0.002 0.004 0.007 0.017] m  valve_area_TLU=[1e-09, 2.0352e-07, 4.0736e-05, .00011438, .00034356] m^2  del_S_flow_TLU=[0 0.002 0.004 0.007 0.017] m  p_diff_TLU=[-.1, .3, .5, .7] MPa  vol_flow_TLU=[-1e-08, 2.2e-08, 2.8e-08, 3.4e-08; -9e-06, .00015, .0002, .00024; -.00036, .00063, .00081, .00096; -.00054, .00094, .0012, .0014; -.00091, .0016, .002, .0024] m^3/s  mdot_TLU=[-1e-05, 1.7e-05, 2e-05, 2.6e-05; -.002, .0035, .0045, .0053; -.4, .7, .9, 1.06; -1.13, 1.96, 2.5, 3; -3.45, 6, 7.7, 9.13] kg/s  p_diff_TLU_const=[-.1, .3, .5, .7] MPa  vol_flow_TLU_const=[-.0009, .0016, .002, .0024] m^3/s  mdot_TLU_const=[-.9, 1.6, 2, 2.4] kg/s  area_const=1e-4 m^2  T_ref_in=293.15 K  p_ref_in=0.101325 MPa  area_leak=pi * (PlntThrValDratioMin*PlntThrPipeDia)^2 / 4 m^2  area=pi * PlntThrPipeDia^2 / 4 m^2  Cd=0.7  Re_c=12  smoothing_factor=0.01  pressure_recovery=simscape.enum.onoff.on  S_max_PA=PlntThrValSplMax m  del_S_max_PA=coolant_valve_displacement-(coolant_valve_displacement)*(pi * (coolant_valve_D_ratio_min*coolant_pipe_D)^2 / 4)/(pi * (coolant_valve_D_ratio_max*coolant_pipe_D)^2 / 4) m  area_max_PA=pi * (coolant_valve_D_ratio_max*coolant_pipe_D)^2 / 4 m^2  del_S_TLU_PA=[0 0.002 0.004 0.007 0.017] m  valve_area_TLU_PA=[1e-09, 2.0352e-07, 4.0736e-05, .00011438, .00034356] m^2  del_S_flow_TLU_PA=[0 0.002 0.004 0.007 0.017] m  p_diff_TLU_PA=[-.1, .3, .5, .7] MPa  vol_flow_TLU_PA=[-1e-08, 2.2e-08, 2.8e-08, 3.4e-08; -9e-06, .00015, .0002, .00024; -.00036, .00063, .00081, .00096; -.00054, .00094, .0012, .0014; -.00091, .0016, .002, .0024] m^3/s  mdot_TLU_PA=[-1e-05, 1.7e-05, 2e-05, 2.6e-05; -.002, .0035, .0045, .0053; -.4, .7, .9, 1.06; -1.13, 1.96, 2.5, 3; -3.45, 6, 7.7, 9.13] kg/s  area_const_PA=1e-4 m^2  p_diff_TLU_const_PA=[-.1, .3, .5, .7] MPa  vol_flow_TLU_const_PA=[-.0009, .0016, .002, .0024] m^3/s  mdot_TLU_const_PA=[-.9, 1.6, 2, 2.4] kg/s  S_max_PB=-PlntThrValSplMax m  del_S_max_PB=coolant_valve_displacement-(coolant_valve_displacement)*(pi * (coolant_valve_D_ratio_min*coolant_pipe_D)^2 / 4)/(pi * (coolant_valve_D_ratio_max*coolant_pipe_D)^2 / 4) m  area_max_PB=pi * (coolant_valve_D_ratio_max*coolant_pipe_D)^2 / 4 m^2  del_S_TLU_PB=[0 0.002 0.004 0.007 0.017] m  valve_area_TLU_PB=[1e-09, 2.0352e-07, 4.0736e-05, .00011438, .00034356] m^2  del_S_flow_TLU_PB=[0 0.002 0.004 0.007 0.017] m  p_diff_TLU_PB=[-.1, .3, .5, .7] MPa  vol_flow_TLU_PB=[-1e-08, 2.2e-08, 2.8e-08, 3.4e-08; -9e-06, .00015, .0002, .00024; -.00036, .00063, .00081, .00096; -.00054, .00094, .0012, .0014; -.00091, .0016, .002, .0024] m^3/s  mdot_TLU_PB=[-1e-05, 1.7e-05, 2e-05, 2.6e-05; -.002, .0035, .0045, .0053; -.4, .7, .9, 1.06; -1.13, 1.96, 2.5, 3; -3.45, 6, 7.7, 9.13] kg/s  area_const_PB=1e-4 m^2  p_diff_TLU_const_PB=[-.1, .3, .5, .7] MPa  vol_flow_TLU_const_PB=[-.0009, .0016, .002, .0024] m^3/s  mdot_TLU_const_PB=[-.9, 1.6, 2, 2.4] kg/s  S_max_AB=7.5e-3 m  del_S_max_AB=0.005 m  area_max_AB=1e-4 m^2  del_S_TLU_AB=[0, .00125, .0025, .00375, .005] m  valve_area_TLU_AB=[1e-10, 1e-05, 4e-05, 6e-05, .0001] m^2  del_S_flow_TLU_AB=[0, .00125, .0025, .00375, .005] m  p_diff_TLU_AB=[-.1, .3, .5, .7] MPa  vol_flow_TLU_AB=[-1e-08, 2.2e-08, 2.8e-08, 3.4e-08; -9e-06, .00015, .0002, .00024; -.00036, .00063, .00081, .00096; -.00054, .00094, .0012, .0014; -.00091, .0016, .002, .0024] m^3/s  mdot_TLU_AB=[1.7e-05, 2e-05, 2.6e-05; .0035, .0045, .0053; .7, .9, 1.06; 1.96, 2.5, 3; 6, 7.7, 9.13] kg/s  area_const_AB=1e-4 m^2  p_diff_TLU_const_AB=[-.1, .3, .5, .7] MPa  vol_flow_TLU_const_AB=[-.0009, .0016, .002, .0024] m^3/s  mdot_TLU_const_AB=[-.9, 1.6, 2, 2.4] kg/s  S_max_AT=-PlntThrValSplMax m  del_S_max_AT=coolant_valve_displacement-(coolant_valve_displacement)*(pi * (coolant_valve_D_ratio_min*coolant_pipe_D)^2 / 4)/(pi * (coolant_valve_D_ratio_max*coolant_pipe_D)^2 / 4) m  area_max_AT=pi * (coolant_valve_D_ratio_max*coolant_pipe_D)^2 / 4 m^2  del_S_TLU_AT=[0 0.002 0.004 0.007 0.017] m  valve_area_TLU_AT=[1e-09, 2.0352e-07, 4.0736e-05, .00011438, .00034356] m^2  del_S_flow_TLU_AT=[0 0.002 0.004 0.007 0.017] m  p_diff_TLU_AT=[-.1, .3, .5, .7] MPa  vol_flow_TLU_AT=[-1e-08, 2.2e-08, 2.8e-08, 3.4e-08; -9e-06, .00015, .0002, .00024; -.00036, .00063, .00081, .00096; -.00054, .00094, .0012, .0014; -.00091, .0016, .002, .0024] m^3/s  mdot_TLU_AT=[-1e-05, 1.7e-05, 2e-05, 2.6e-05; -.002, .0035, .0045, .0053; -.4, .7, .9, 1.06; -1.13, 1.96, 2.5, 3; -3.45, 6, 7.7, 9.13] kg/s  area_const_AT=1e-4 m^2  p_diff_TLU_const_AT=[-.1, .3, .5, .7] MPa  vol_flow_TLU_const_AT=[-.0009, .0016, .002, .0024] m^3/s  mdot_TLU_const_AT=[-.9, 1.6, 2, 2.4] kg/s  S_max_BT=PlntThrValSplMax m  del_S_max_BT=coolant_valve_displacement-(coolant_valve_displacement)*(pi * (coolant_valve_D_ratio_min*coolant_pipe_D)^2 / 4)/(pi * (coolant_valve_D_ratio_max*coolant_pipe_D)^2 / 4) m  area_max_BT=pi * (coolant_valve_D_ratio_max*coolant_pipe_D)^2 / 4 m^2  del_S_TLU_BT=[0 0.002 0.004 0.007 0.017] m  valve_area_TLU_BT=[1e-09, 2.0352e-07, 4.0736e-05, .00011438, .00034356] m^2  del_S_flow_TLU_BT=[0 0.002 0.004 0.007 0.017] m  p_diff_TLU_BT=[-.1, .3, .5, .7] MPa  vol_flow_TLU_BT=[-1e-08, 2.2e-08, 2.8e-08, 3.4e-08; -9e-06, .00015, .0002, .00024; -.00036, .00063, .00081, .00096; -.00054, .00094, .0012, .0014; -.00091, .0016, .002, .0024] m^3/s  mdot_TLU_BT=[-1e-05, 1.7e-05, 2e-05, 2.6e-05; -.002, .0035, .0045, .0053; -.4, .7, .9, 1.06; -1.13, 1.96, 2.5, 3; -3.45, 6, 7.7, 9.13] kg/s  area_const_BT=1e-4 m^2  p_diff_TLU_const_BT=[-.1, .3, .5, .7] MPa  vol_flow_TLU_const_BT=[-.0009, .0016, .002, .0024] m^3/s  mdot_TLU_const_BT=[-.9, 1.6, 2, 2.4] kg/s  S_max_PT=0 m  del_S_max_PT=0.005 m  area_max_PT=1e-4 m^2  del_S_TLU_PT=[0, .00125, .0025, .00375, .005] m  valve_area_TLU_PT=[1e-10, 1e-05, 4e-05, 6e-05, .0001] m^2  del_S_flow_TLU_PT=[0, .00125, .0025, .00375, .005] m  p_diff_TLU_PT=[-.1, .3, .5, .7] MPa  vol_flow_TLU_PT=[-1e-08, 2.2e-08, 2.8e-08, 3.4e-08; -9e-06, .00015, .0002, .00024; -.00036, .00063, .00081, .00096; -.00054, .00094, .0012, .0014; -.00091, .0016, .002, .0024] m^3/s  mdot_TLU_PT=[1.7e-05, 2e-05, 2.6e-05; .0035, .0045, .0053; .7, .9, 1.06; 1.96, 2.5, 3; 6, 7.7, 9.13] kg/s
  Battery Coolant Tank : SimscapeFluids_lib/Thermal Liquid/Tanks & Accumulators/Tank (G-TL)  num_inlet=2  volume_total=PlntThrTankVol l  volume_spec=1  tank_area=PlntThrTankArea m^2  level_TLU=[0, 3, 5] m  volume_TLU=[0, 4, 6] m^3  inlet_areas_A1B1=[.01, .01] m^2  inlet_height_A2=0.1 m  inlet_area_A2=0.01 m^2  inlet_heights_A2B2=[0, 0] m  inlet_areas_A2B2=[1 1] * pi * PlntThrPipeDia^2 / 4 m^2  inlet_heights_A2B2C2=[.1, .1, .1] m  inlet_areas_A2B2C2=[.01, .01, .01] m^2  inlet_heights_A2B2C2D2=0.1 * ones(1, 4) m  inlet_areas_A2B2C2D2=0.01 * ones(1, 4) m^2  inlet_heights_A2B2C2D2E2=0.1 * ones(1, 5) m  inlet_areas_A2B2C2D2E2=0.01 * ones(1, 5) m^2  inlet_heights_A2B2C2D2E2F2=0.1 * ones(1, 6) m  inlet_areas_A2B2C2D2E2F2=0.01 * ones(1, 6) m^2  capacity_check=0  max_liquid_capacity=coolant_tank_volume l  g=0 m/s^2  level_specify=on  level_priority=None  level=0.15 m  level_nominal_specify=off  level_nominal_value=1  level_nominal_unit=m  volume_liquid_specify=on  volume_liquid_priority=High  volume_liquid=0.5 * PlntThrTankVol l  volume_liquid_nominal_specify=off  volume_liquid_nominal_value=1  volume_liquid_nominal_unit=m^3  mass_liquid_specify=off  mass_liquid_priority=None  mass_liquid=5e+3 kg  mass_liquid_nominal_specify=off  mass_liquid_nominal_value=1  mass_liquid_nominal_unit=kg  T_liquid_specify=on  T_liquid_priority=High  T_liquid=EnvAirTemp K  T_liquid_nominal_specify=off  T_liquid_nominal_value=1  T_liquid_nominal_unit=K  p_gas_specify=on  p_gas_priority=High  p_gas=EnvAbsPrs Pa  p_gas_nominal_specify=off  p_gas_nominal_value=1  p_gas_nominal_unit=MPa  T_gas_specify=on  T_gas_priority=High  T_gas=EnvAirTemp K  T_gas_nominal_specify=off  T_gas_nominal_value=1  T_gas_nominal_unit=K  rho_gas_specify=off  rho_gas_priority=None  rho_gas=1.2 kg/m^3  rho_gas_nominal_specify=off  rho_gas_nominal_value=1  rho_gas_nominal_unit=kg/m^3
  Battery Coolant Tank Heat Transfer : Subsystem
  Bias : Bias  Bias=-1
  Cap (G){,1..3} (4 alike) : fl_lib/Gas/Elements/Cap (G)  p_specify=off  p_priority=None  p=0.101325 MPa  p_nominal_specify=off  p_nominal_value=1  p_nominal_unit=MPa  T_specify=off  T_priority=None  T=293.15 K  T_nominal_specify=off  T_nominal_value=1  T_nominal_unit=K
  Coolant Properties : SimscapeFluids_lib/Thermal Liquid/Utilities/Thermal Liquid Properties (TL)  fluid_list=fluids.thermal_liquid.utilities.enum.thermal_liquid_fluid_list.ethylene_glycol  concentration_param_EG=fluids.thermal_liquid.utilities.enum.thermal_liquid_concentration.volume_fraction  concentration_param_PG=fluids.thermal_liquid.utilities.enum.thermal_liquid_concentration.volume_fraction  c_mass_SW=3.5e-3  c_mass_EG=0.1  c_mass_PG=0.1  c_mass_GL=0.1  c_vol_EG=0.5  c_vol_PG=0.1  beta_const_EG=2.1791 GPa  beta_const_PG=2.1791 GPa  beta_const_GL=2.1791 GPa  p_min_EG=0.01 MPa  p_min_PG=0.01 MPa  p_min_GL=0.01 MPa  p_max_EG=50 MPa  p_max_PG=50 MPa  p_max_GL=50 MPa  p_atm=0.101325 MPa  properties_range_check=simscape.enum.assert.action.error
  Gain : Gain  Gain=2
  LPF with IC1 : Subsystem  mask{wc=1, InitCond=0, dataType=off}
      mask prompts: wc "Cutoff frequency, wc [rad/s]"; InitCond "Initial condition, InitCond [same as u]"; dataType "Enforce same input data type"
  Max Valve Displacement [m] : Gain  Gain=PlntThrValDisp
  Motor Coolant Tank : SimscapeFluids_lib/Thermal Liquid/Tanks & Accumulators/Tank (G-TL)  num_inlet=2  volume_total=PlntThrTankVol l  volume_spec=1  tank_area=PlntThrTankArea m^2  level_TLU=[0, 3, 5] m  volume_TLU=[0, 4, 6] m^3  inlet_areas_A1B1=[.01, .01] m^2  inlet_height_A2=0.1 m  inlet_area_A2=0.01 m^2  inlet_heights_A2B2=[0, 0] m  inlet_areas_A2B2=[1 1] * PlntThrPipeArea m^2  inlet_heights_A2B2C2=[.1, .1, .1] m  inlet_areas_A2B2C2=[.01, .01, .01] m^2  inlet_heights_A2B2C2D2=0.1 * ones(1, 4) m  inlet_areas_A2B2C2D2=0.01 * ones(1, 4) m^2  inlet_heights_A2B2C2D2E2=0.1 * ones(1, 5) m  inlet_areas_A2B2C2D2E2=0.01 * ones(1, 5) m^2  inlet_heights_A2B2C2D2E2F2=0.1 * ones(1, 6) m  inlet_areas_A2B2C2D2E2F2=0.01 * ones(1, 6) m^2  capacity_check=0  max_liquid_capacity=coolant_tank_volume l  g=0 m/s^2  level_specify=on  level_priority=None  level=0.15 m  level_nominal_specify=off  level_nominal_value=1  level_nominal_unit=m  volume_liquid_specify=on  volume_liquid_priority=High  volume_liquid=0.5*PlntThrTankVol l  volume_liquid_nominal_specify=off  volume_liquid_nominal_value=1  volume_liquid_nominal_unit=m^3  mass_liquid_specify=off  mass_liquid_priority=None  mass_liquid=5e+3 kg  mass_liquid_nominal_specify=off  mass_liquid_nominal_value=1  mass_liquid_nominal_unit=kg  T_liquid_specify=on  T_liquid_priority=High  T_liquid=EnvAirTemp K  T_liquid_nominal_specify=off  T_liquid_nominal_value=1  T_liquid_nominal_unit=K  p_gas_specify=on  p_gas_priority=High  p_gas=EnvAbsPrs Pa  p_gas_nominal_specify=off  p_gas_nominal_value=1  p_gas_nominal_unit=MPa  T_gas_specify=on  T_gas_priority=High  T_gas=EnvAirTemp K  T_gas_nominal_specify=off  T_gas_nominal_value=1  T_gas_nominal_unit=K  rho_gas_specify=off  rho_gas_priority=None  rho_gas=1.2 kg/m^3  rho_gas_nominal_specify=off  rho_gas_nominal_value=1  rho_gas_nominal_unit=kg/m^3
  Motor Coolant Tank Heat Transfer : Subsystem
  Simulink-PS Converter : nesl_utility/Simulink-PS Converter  PhysicalDomain=network_engine_domain  SubClassName=ps_input  LeftPortType=input  RightPortType=output  PseudoPeriodic=off  Frequencies=[]  NoiseDistribution=none  NoiseParameters=[]  Unit=m  AffineConversion=off  FilteringAndDerivatives=provide  SimscapeFilterOrder=1  InputFilterTimeConstant=0.001  UdotUserProvided=0
  D : PMIOPort  Side=Left
  A : PMIOPort  Port=2  Side=Left
  B : PMIOPort  Port=3  Side=Right
  C : PMIOPort  Port=4  Side=Right
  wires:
  [AmbTemp] -> Battery Coolant Tank Heat Transfer/1(AmbTemp)
  1/1 -> Motor Coolant Tank Heat Transfer/1(AmbTemp), [AmbTemp]
  Gain/1 -> Bias/1
  Bias/1 -> Max Valve Displacement [m]/1
  Max Valve Displacement [m]/1 -> Simulink-PS Converter/1
  2/1 -> LPF with IC1/1(u)
  LPF with IC1/1(y) -> Gain/1
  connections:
  4-Way Valve/RConn3 -- Coolant Properties/RConn1 -- C/RConn1
  4-Way Valve/RConn1 -- Simulink-PS Converter/RConn1
  4-Way Valve/LConn2 -- Motor Coolant Tank/LConn3
  Cap (G)1/LConn1 -- Motor Coolant Tank/LConn2
  Cap (G)/LConn1 -- Motor Coolant Tank/LConn1
  Motor Coolant Tank Heat Transfer/RConn1 -- Motor Coolant Tank/RConn1
  Motor Coolant Tank Heat Transfer/RConn2 -- Motor Coolant Tank/RConn2
  D/RConn1 -- Motor Coolant Tank/LConn4
  Cap (G)2/LConn1 -- Battery Coolant Tank/LConn1
  Cap (G)3/LConn1 -- Battery Coolant Tank/LConn2
  B/RConn1 -- Battery Coolant Tank/LConn4
  4-Way Valve/LConn1 -- Battery Coolant Tank/LConn3
  Battery Coolant Tank Heat Transfer/LConn1 -- Battery Coolant Tank/RConn1
  Battery Coolant Tank Heat Transfer/LConn2 -- Battery Coolant Tank/RConn2
  4-Way Valve/RConn2 -- A/RConn1
